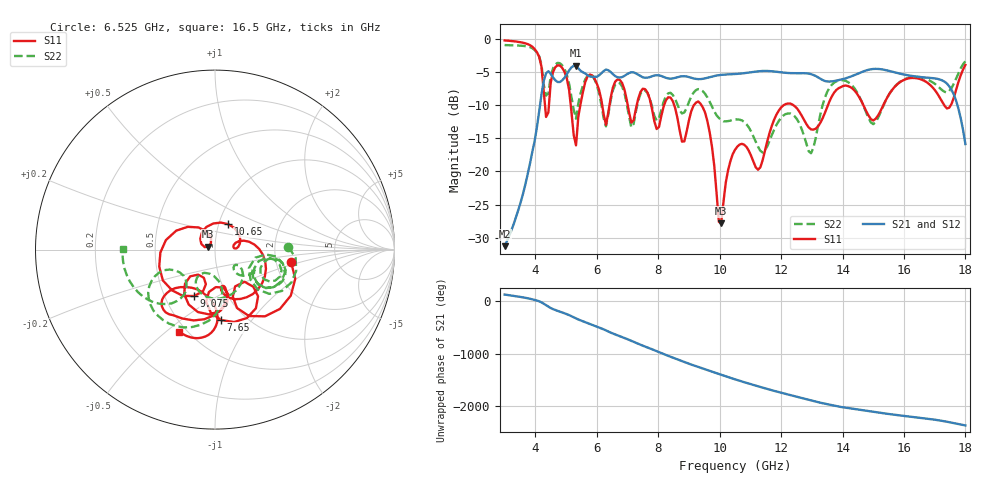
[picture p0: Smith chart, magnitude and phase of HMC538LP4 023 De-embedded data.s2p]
! Chelmsford, MA 01824
! http://www.hittite.com
! Tel: 978-250-3343
! Fax: 978-250-3373
! Device  :  HMC538LP4
! Description:  600 Analog Phase Shifter
! Frequency  :  6.0 GHz - 15.0 GHz
! Package  :  LP4  - 4x4 mm Quad Flatpack No-Lead (QFN) Plastic Package: 24 pin
! Ports  :  2 RF, 1 DC
!  Pin  3  = Rfin  = Port 1
!  Pin  16  = Rfout = Port 2
!  pin  21  = vCTL
! Voltages:  VCTL  = 0 to 5.0 Volts
! Currents :  Vb(V)  Vd(V)  Ib(mA)  Id(mA)
!  0.00  2.30  0.000000	0.471374
! Data:  The device was measured on evaluation board 111296-1.
!  Data was collected using a calibrated network analyzer.
!  The evaluation circuit board was modeled and simulated.This was use
!  to removed the evaluation board circuit from the measured data.
!  The reference plane is the center of the package pin.
! Misc:  Lot #
!Date Measured:  03 - 11 -2009
! Date:  03 - 17 -2009
! Note:
!  Hittite Microwave supplies this data as a sample of measured data at the
!  package pin for this package product.  Your particular data for this product
!  may vary.
!  Data was taken at 25 degrees C.
!  Hittite Microwave reserves the right to change this data at anytime.
# MHz S MA R 50
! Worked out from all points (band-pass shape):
!   201 points, 3 GHz to 18 GHz, reference 50 ohm
!   highest |S21| = -4.05 dB at 5.325 GHz (marker M1); lowest = -31.3 dB at 3 GHz (marker M2)
!   |S21| within 3 dB of the highest: 4.248 GHz to 17.46 GHz (13.21 GHz wide, 122 % of centre)
!   lowest |S11| = -27.8 dB at 10.05 GHz (marker M3), VSWR 1.08, Z = 46.4 + j1.59 ohm
!   |S11| at or under -10 dB: 8.521 GHz to 9.162 GHz (641 MHz wide, 7.25 % of centre); 9.407 GHz to 12.08 GHz (2.677 GHz wide, 24.9 % of centre); 12.4 GHz to 13.52 GHz (1.127 GHz wide, 8.7 % of centre)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
!   |S22| runs from -17.2 to -0.9 dB; largest |S21 - S12| = 0.003
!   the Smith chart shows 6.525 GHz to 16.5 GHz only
!   S11 on the Smith chart (normalised r, x): 6.525 GHz: 2.42, -0.41; 7.65 GHz: 0.78, -0.72; 9.075 GHz: 0.70, -0.39; 10.65 GHz: 1.11, +0.32; 16.5 GHz: 0.45, -0.56
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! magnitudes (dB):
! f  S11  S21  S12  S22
! 3 GHz  -0.2  -31.3  -31.3  -0.9
! 4.05 GHz  -2.0  -13.4  -13.3  -2.0
! 4.35 GHz  -11.8  -5.2  -5.2  -8.6
! 4.8 GHz  -4.0  -6.5  -6.5  -3.7
! 5.325 GHz  -16.1  -4.1  -4.1  -12.0
! 5.55 GHz  -8.0  -5.1  -5.1  -7.0
! 6.3 GHz  -13.0  -4.6  -4.6  -13.2
! 6.525 GHz  -7.3  -5.3  -5.3  -7.8
! 7.125 GHz  -12.6  -5.0  -5.0  -13.3
! 7.65 GHz  -8.1  -5.8  -5.9  -8.2
! 8.025 GHz  -13.3  -5.5  -5.5  -12.0
! 9.075 GHz  -10.9  -5.9  -5.9  -8.7
! 9.6 GHz  -12.4  -5.9  -5.9  -8.8
! 10.05 GHz  -27.8  -5.4  -5.4  -12.2
! 10.5 GHz  -16.7  -5.3  -5.3  -12.1
! 10.65 GHz  -15.9  -5.3  -5.3  -12.2
! 13.05 GHz  -13.7  -5.4  -5.5  -16.5
! 13.72 GHz  -8.1  -6.4  -6.4  -6.6
! 15.53 GHz  -8.3  -4.8  -4.9  -8.3
! 16.5 GHz  -6.0  -5.7  -5.8  -5.8
! 17.4 GHz  -10.5  -6.7  -6.8  -8.1
! 18 GHz  -3.9  -15.9  -15.9  -3.4
